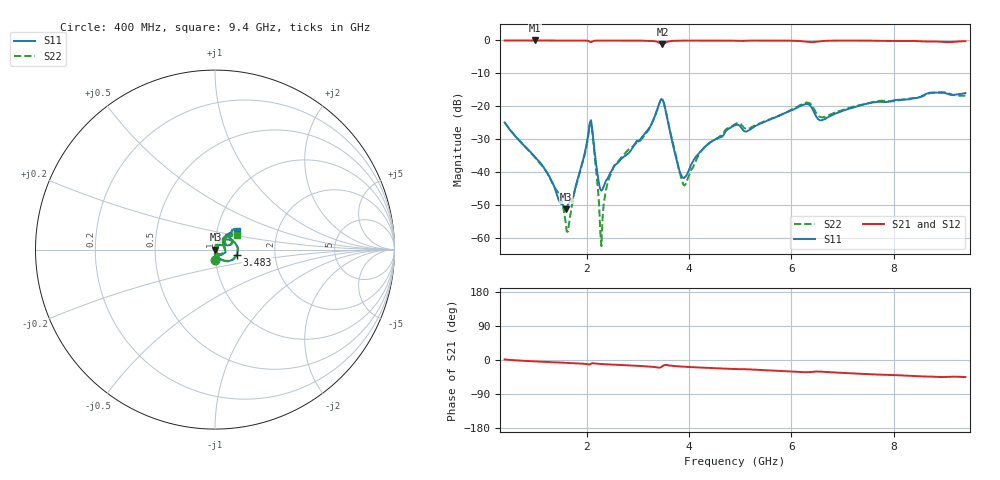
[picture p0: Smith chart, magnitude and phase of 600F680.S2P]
!  American Technical Ceramics  Date:  11/23/05
!  One Norden Lane
!  Huntington Station,  NY.  11746-2102
!  Tel:  (631) 622-4700  Fax:  (631) 622-4748
!  Part Number  600F680  Mounting Orientation: Horizontal
!  Description: Ultra Low ESR Microwave capacitors
!  Application: Coupling, Bypass, Tuning, DC Block
!  Filters, Matching
# GHZ S DB R 50
! Freq  |S11|  S11 Ph  |S21|  S21 Ph  |S12|  S12 Ph  |S22|  S22 Ph
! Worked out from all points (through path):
!   401 points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, 400 MHz to 9.4 GHz, reference 50 ohm
!   highest |S21| = 0.00 dB at 985 MHz (marker M1); lowest = -1.2 dB at 3.483 GHz (marker M2)
!   group delay of S21, straight-line fit = 14.1 ps
!   lowest |S11| = -51.4 dB at 1.593 GHz (marker M3), VSWR 1.01, Z = 50.3 - j0.064 ohm
!   |S11| at or under -10 dB: start of sweep to end of sweep
!   |S22| runs from -62.6 to -15.7 dB; largest |S21 - S12| = 0.0024
!   S11 on the Smith chart (normalised r, x): 400 MHz: 1.00, -0.11; 3.483 GHz: 1.28, -0.08; 9.4 GHz: 1.24, +0.26
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0.4  -24.93 -87.9  -0.02 1.4  -0.01 1.4  -24.91 -88.3
0.985  -35.29 -90.2  0.00 -3.6  -0.01 -3.7  -35.45 -93.9
1.458  -48.58 -64.4  -0.01 -6.6  -0.01 -6.7  -46.45 -88.4
1.593  -51.40 -13.7  -0.01 -7.4  -0.01 -7.5  -55.44 -135.2
1.66  -49.33 14.6  -0.01 -7.8  -0.01 -7.9  -55.56 114.4
1.908  -37.73 61.1  -0.03 -9.6  -0.03 -9.6  -37.94 80.5
2.088  -24.26 -13.7  -0.53 -9.7  -0.53 -9.7  -24.91 -6.0
2.245  -43.73 -42.7  -0.04 -10.2  -0.04 -10.3  -49.78 -71.8
2.29  -45.71 -9.5  -0.03 -10.6  -0.03 -10.7  -62.58 43.8
2.403  -42.25 31.6  -0.02 -11.5  -0.03 -11.5  -43.91 89.1
2.515  -38.94 44.8  -0.03 -12.2  -0.03 -12.3  -38.88 86.9
3.168  -27.80 58.8  -0.10 -16.7  -0.10 -16.7  -28.19 59.5
3.415  -19.40 28.2  -0.65 -20.1  -0.65 -20.1  -19.44 30.0
3.483  -17.91 -13.4  -1.17 -16.3  -1.17 -16.3  -17.92 -11.0
3.798  -38.76 -46.5  -0.08 -16.8  -0.08 -16.8  -38.68 -54.0
3.91  -41.80 4.1  -0.06 -17.8  -0.05 -17.8  -44.13 0.2
4.27  -33.07 55.1  -0.05 -20.2  -0.05 -20.2  -33.07 65.0
4.9  -25.82 49.9  -0.09 -24.1  -0.09 -24.1  -25.45 55.3
6.408  -20.69 19.0  -0.50 -31.1  -0.51 -31.1  -19.94 19.3
6.588  -24.29 35.1  -0.19 -30.8  -0.19 -30.8  -23.38 29.5
7.915  -18.59 48.7  -0.13 -39.4  -0.13 -39.3  -18.50 38.8
9.4  -16.01 40.5  -0.22 -45.1  -0.23 -45.1  -16.80 33.0
